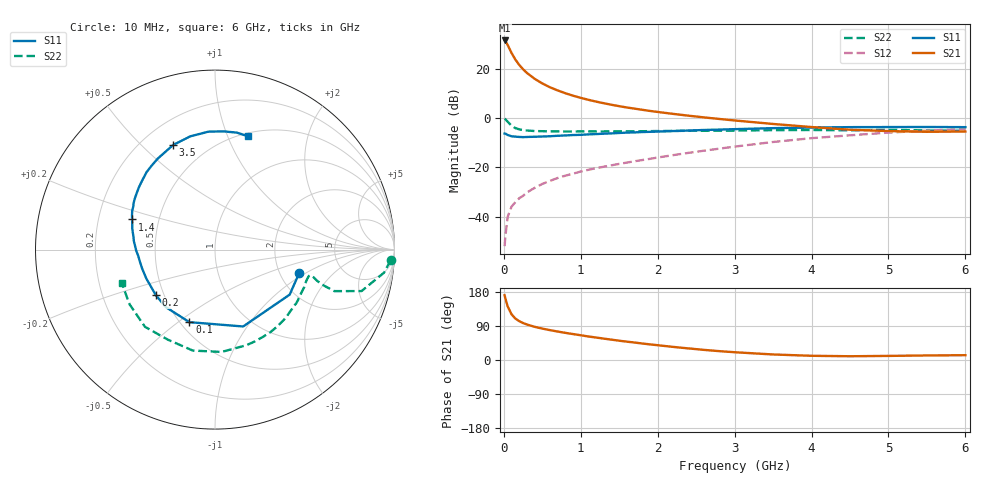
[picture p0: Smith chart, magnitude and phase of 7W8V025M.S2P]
! Infineon Technologies  Discrete & RF Semiconductors
! BFS17W
! Si NPN RF Bipolar Junction Transistor in SOT323
! VCE = 8 V  IC = 25 mA
! Common Emitter S-Parameters:  August  1999
# GHz  S  MA  R  50
!  f  S11  S21  S12  S22
! GHz  MAG  ANG  MAG  ANG  MAG  ANG  MAG  ANG
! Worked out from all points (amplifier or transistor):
!   36 points, 10 MHz to 6 GHz, reference 50 ohm
!   highest |S21| = 31.6 dB at 10 MHz (marker M1)
!   |S21| within 3 dB of that: start of sweep to 67.74 MHz
!   unconditionally stable (mu >= 1): 252.5 MHz to 1.988 GHz; 5.545 GHz to end of sweep
!   at 250 MHz: K = 1.00, MSG = 25.7 dB, |S12| = -31.6 dB
!   at 1.4 GHz: K = 1.13, MAG = 10.1 dB, |S12| = -19.1 dB
!   at 6 GHz: K = 1.03, MAG = -1.6 dB, |S12| = -4.4 dB
!   S11 on the Smith chart (normalised r, x): 10 MHz: 2.55, -0.88; 100 MHz: 0.56, -0.55; 200 MHz: 0.45, -0.28; 1.4 GHz: 0.35, +0.16; 3.5 GHz: 0.33, +0.63; 6 GHz: 0.53, +1.19
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0.01  0.4868 -15.7  38.09 171.1  0.0025 85.1  0.9808 -3.5
0.02  0.4858 -31.1  37.09 162.4  0.004 83.4  0.95 -7.8
0.05  0.4561 -69.9  30.75 141.3  0.0099 68.5  0.8487 -15.8
0.1  0.4287 -109.4  21.24 120.6  0.0159 62.0  0.7034 -19.2
0.15  0.4218 -130.5  15.55 109.3  0.0197 60.4  0.6284 -18.1
0.2  0.416 -142.6  12.13 102.5  0.0236 63.3  0.5931 -16.9
0.25  0.4121 -151.0  9.889 97.5  0.0264 63.7  0.5727 -15.8
0.3  0.4153 -157.0  8.33 93.7  0.0309 66.5  0.562 -15.3
0.4  0.4196 -165.7  6.33 87.6  0.0383 68.3  0.5485 -15.1
0.5  0.4241 -171.2  5.093 82.9  0.0461 70.1  0.5441 -15.6
0.6  0.4296 -175.5  4.249 78.8  0.0531 71.1  0.5411 -16.5
0.7  0.4393 -179.4  3.668 75.1  0.0609 71.7  0.5388 -17.8
0.9  0.4547 174.0  2.868 68.4  0.0746 72.5  0.5365 -21.1
1.1  0.4689 167.9  2.364 62.0  0.0894 73.2  0.538 -24.9
1.4  0.4915 160.0  1.875 53.7  0.1103 74.0  0.5413 -31.3
1.8  0.5229 150.0  1.481 43.5  0.141 75.6  0.5434 -40.8
2.2  0.5481 140.7  1.225 34.6  0.1773 75.8  0.5509 -50.6
2.8  0.5863 126.9  0.965 23.4  0.2402 73.8  0.5576 -66.6
3.5  0.6279 111.8  0.764 14.6  0.3284 68.6  0.5714 -86.3
4.5  0.6582 93.2  0.583 9.9  0.4488 56.1  0.5663 -117.7
5.5  0.663 79.4  0.529 12.0  0.5583 42.8  0.5653 -147.3
6  0.6577 73.8  0.536 12.7  0.6014 36.2  0.5522 -160.6
